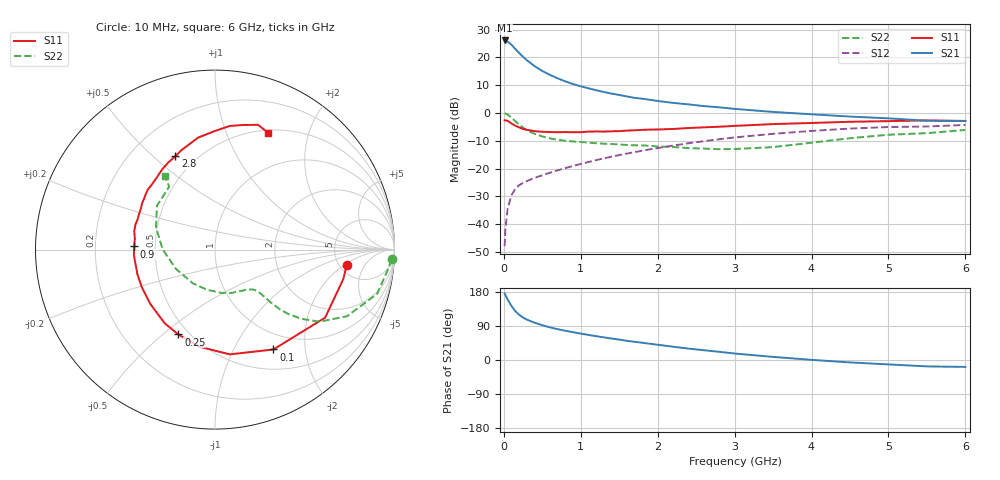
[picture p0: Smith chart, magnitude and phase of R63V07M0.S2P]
! SIEMENS Small Signal Semiconductors
! BFR193
! Si NPN RF Bipolar Junction Transistor in SOT23
! VCE = 3 V  IC = 7 mA
! Common Emitter S-Parameters:  May  1996
# GHz  S  MA  R  50
!  f  S11  S21  S12  S22
! GHz  MAG  ANG  MAG  ANG  MAG  ANG  MAG  ANG
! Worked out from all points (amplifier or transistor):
!   36 points, 10 MHz to 6 GHz, reference 50 ohm
!   highest |S21| = 26.1 dB at 10 MHz (marker M1)
!   |S21| within 3 dB of that: start of sweep to 146.9 MHz
!   unconditionally stable (mu >= 1): 811.3 MHz to 1.869 GHz; 1.965 GHz to 2.019 GHz
!   at 250 MHz: K = 0.53, MSG = 22.7 dB, |S12| = -25.2 dB
!   at 1.4 GHz: K = 1.05, MAG = 10.0 dB, |S12| = -15.8 dB
!   at 6 GHz: K = 0.96, MSG = 0.7 dB, |S12| = -4.3 dB
!   lowest NFmin = 1.20 dB at 450 MHz
!   S11 on the Smith chart (normalised r, x): 10 MHz: 5.80, -2.20; 100 MHz: 0.76, -1.45; 250 MHz: 0.44, -0.57; 900 MHz: 0.38, +0.02; 2.8 GHz: 0.39, +0.59; 6 GHz: 0.53, +1.42
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0.01  0.7388 -6.7  20.2 175.9  0.004 83.6  0.9866 -3.2
0.02  0.7335 -12.9  20.05 171.3  0.0081 86.0  0.9718 -6.2
0.05  0.7214 -31.7  19.19 159.4  0.0192 75.2  0.9368 -15.2
0.1  0.6446 -59.7  16.85 142.3  0.0334 64.4  0.8236 -26.8
0.15  0.5896 -81.9  14.14 128.8  0.0433 57.3  0.7075 -34.6
0.2  0.5479 -99.3  12.02 119.3  0.0504 53.6  0.617 -38.7
0.25  0.515 -113.3  10.26 111.9  0.055 51.8  0.543 -41.3
0.3  0.4971 -124.3  8.886 106.4  0.0595 51.6  0.4893 -42.7
0.4  0.4704 -140.3  6.976 98.4  0.068 51.7  0.4214 -43.5
0.5  0.4585 -152.7  5.695 91.7  0.0755 53.1  0.3776 -43.7
0.6  0.4537 -162.2  4.841 86.1  0.0841 54.9  0.3482 -44.0
0.7  0.4501 -170.1  4.199 81.3  0.0927 56.5  0.3294 -44.6
0.9  0.4501 177.8  3.312 73.3  0.1113 58.4  0.307 -46.4
1.1  0.4615 167.3  2.776 66.2  0.131 59.7  0.2925 -49.9
1.3  0.4628 158.7  2.382 59.8  0.1525 60.3  0.2791 -53.5
1.6  0.4812 147.7  1.98 50.6  0.1858 59.5  0.2653 -61.5
2.2  0.5153 129.2  1.518 35.0  0.2589 55.5  0.2442 -81.7
2.8  0.5653 113.0  1.264 21.6  0.3364 48.4  0.2226 -111.6
3.5  0.6305 98.7  1.044 8.2  0.4211 37.9  0.2429 -153.8
4.5  0.6938 83.2  0.861 -6.4  0.5236 22.1  0.3512 159.4
5.5  0.7352 71.0  0.725 -16.9  0.5708 5.8  0.4334 126.1
6  0.7159 65.6  0.72 -18.2  0.6084 1.1  0.4946 124.2
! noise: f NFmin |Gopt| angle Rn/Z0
0.45  1.2  0.24  125  0.12
0.9  1.25  0.36  154  0.11
1.8  2  0.55  -156  0.13
